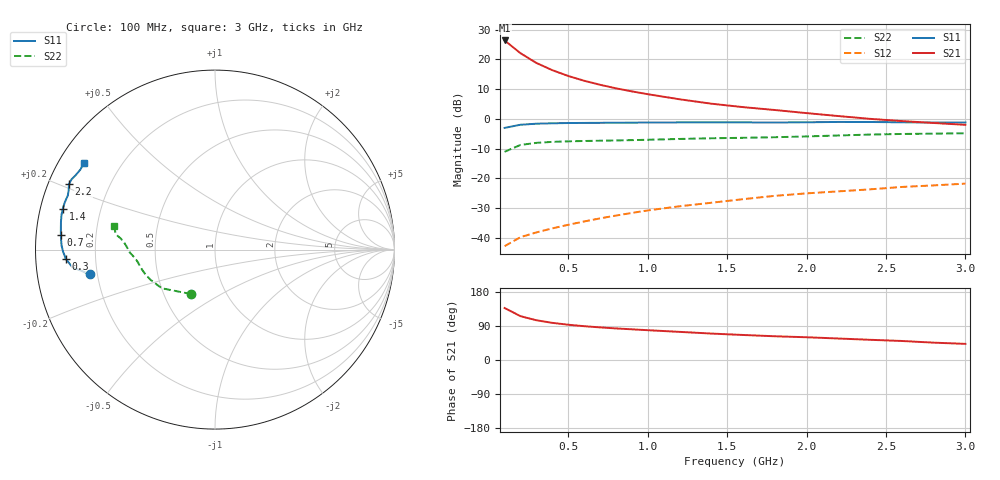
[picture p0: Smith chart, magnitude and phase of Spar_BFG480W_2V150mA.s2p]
! Filename: 2150BFG480.001
! Title: BFG480W
! Bias: Vce=2V; Ic=150mA
! Company: NXP Semiconductors NL
! User: Quality&Reliability T&D
! Measure time: 10 Nov 1999 / 11:55:59
#  MHz  S  MA  R 50
! Freq  S11  S21  S12  S22  :
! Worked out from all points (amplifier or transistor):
!   20 points, 100 MHz to 3 GHz, reference 50 ohm
!   highest |S21| = 26.4 dB at 100 MHz (marker M1)
!   |S21| within 3 dB of that: start of sweep to 169.9 MHz
!   unconditionally stable (mu >= 1): start of sweep to end of sweep
!   at 400 MHz: K = 1.53, MAG = 22.3 dB, |S12| = -36.8 dB
!   at 1.2 GHz: K = 1.65, MAG = 13.3 dB, |S12| = -29.3 dB
!   at 3 GHz: K = 1.69, MAG = 5.0 dB, |S12| = -21.7 dB
!   S11 on the Smith chart (normalised r, x): 100 MHz: 0.17, -0.10; 300 MHz: 0.09, -0.03; 700 MHz: 0.07, +0.05; 1.4 GHz: 0.07, +0.13; 2.2 GHz: 0.06, +0.21; 3 GHz: 0.07, +0.30
100  0.7083 -168.8  20.89 137.2  0.007285 56.5  0.2812 -118.3
200  0.8004 -172.9  12.75 115.6  0.01032 52.5  0.3664 -144.0
300  0.8333 -176.5  8.741 104.8  0.01241 55.1  0.3971 -155.0
400  0.8468 -179.3  6.618 98.1  0.01451 58.5  0.4124 -160.9
500  0.855 178.5  5.284 93.1  0.01665 61.6  0.4211 -164.5
600  0.859 176.5  4.397 89.2  0.01894 63.8  0.4269 -167.0
700  0.8623 174.7  3.762 86.1  0.02134 66.2  0.4313 -169.0
800  0.8653 173.1  3.282 83.3  0.0238 67.9  0.4356 -170.8
900  0.8681 171.5  2.913 81.0  0.02635 69.6  0.4412 -172.3
1000  0.8715 170.0  2.613 78.7  0.02901 70.5  0.4474 -173.8
1200  0.8768 167.3  2.147 74.3  0.0341 71.9  0.4617 -176.1
1400  0.8778 164.9  1.809 69.8  0.03907 72.5  0.4742 -177.9
1600  0.8773 162.4  1.584 66.1  0.04489 73.0  0.4829 -179.8
1800  0.8735 159.8  1.417 62.6  0.05108 73.1  0.4936 177.8
2000  0.8801 157.8  1.255 60.0  0.05624 73.7  0.509 175.4
2200  0.8918 155.9  1.121 56.7  0.0607 73.5  0.5283 173.3
2400  0.8901 153.9  1.005 53.3  0.06569 72.8  0.547 172.0
2600  0.8796 151.8  0.9227 50.2  0.07207 71.8  0.5601 170.9
2800  0.8724 149.2  0.8565 45.8  0.07652 70.2  0.567 169.3
3000  0.8756 146.5  0.7981 42.6  0.08198 69.3  0.576 166.8
